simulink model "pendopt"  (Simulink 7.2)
settings: Solver=ode3  StartTime=0.0  StopTime=10  FixedStep=0.1  RelTol=1e-3
PreLoadFcn:
  | pid=readfis('pid.fis');
undefined symbols (not defined in the file or in its folder): d_val, deg, i_val, kg, m, N, p_val, s
libraries: mblibv1 x8, simulink_extras x1

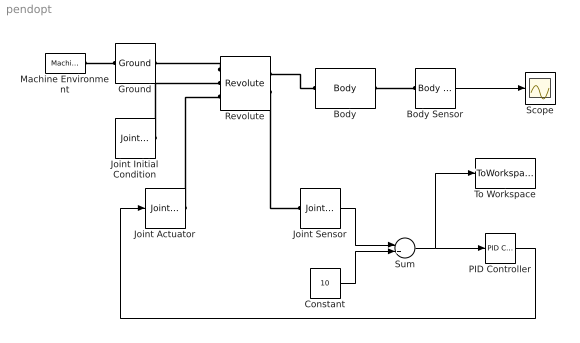
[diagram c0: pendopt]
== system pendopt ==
  Body : mblibv1/Bodies/Body  DialogController=MECH.DynMechDlgSource  PhysicalDomain=mechanical  SubClassName=Unknown  LeftPortType=workingframe  RightPortType=workingframe  LConnTagsString=CS1  RConnTagsString=CS2  UpdateFromCAD=off  DialogClass=MechanicalBodyBlock  Mass=1  MassUnits=kg  InertiaUnits=kg*m^2  Inertia=eye(3)  Shape=Cylinder  ShapeDims=[1 1]  ShapeUnits=m  ShapeUse=false  Density=1  DensityUnits=kg/m^3  DensityUse=false  GraphicsMode=MACHINE_DEFAULT  BodyColorSelMode=MACHINE_DEFAULT  BodyColor=[1 0 0]  AttachedToCS=CG  CG=Left$CG$[0 -1 0]$WORLD$WORLD$m$[0 0 0]$Euler X-Y-Z$deg$WORLD$false$none  WorkingFrames=Left$CS1$[0 0 0]$World$World$m$[0 0 0]$Euler X-Y-Z$deg$WORLD$true$none#Right$CS2$[0 -2 0]$World$World$m$[0 0 0]$Euler X-Y-Z$deg$WORLD$true$none  CGPos=[0 -1 0]  CGRot=[0 0 0]  CS0Pos=[]  CS0Rot=[]  CS1Pos=[0 0 0]  CS1Rot=[0 0 0]  CS2Pos=[0 -2 0]  CS2Rot=[0 0 0]  CS3Pos=[]  CS3Rot=[]  CS4Pos=[]  CS4Rot=[]  CS5Pos=[]  CS5Rot=[]  CS6Pos=[]  CS6Rot=[]  CS7Pos=[]  CS7Rot=[]  CS8Pos=[]  CS8Rot=[]  CS9Pos=[]  CS9Rot=[]  CS10Pos=[]  CS10Rot=[]  CS11Pos=[]  CS11Rot=[]  CS12Pos=[]  CS12Rot=[]  CS13Pos=[]  CS13Rot=[]  CS14Pos=[]  CS14Rot=[]  CS15Pos=[]  CS15Rot=[]  CS16Pos=[]  CS16Rot=[]  CS17Pos=[]  CS17Rot=[]  CS18Pos=[]  CS18Rot=[]  CS19Pos=[]  CS19Rot=[]  CS20Pos=[]  CS20Rot=[]
  Body Sensor : mblibv1/Sensors &  Actuators/Body Sensor  DialogController=MECH.DynMechDlgSource  SystemSampleTime=-1  UpdateFromCAD=off  PhysicalDomain=Mechanical  PortType=blob  Muxed=on  Pose=off  Angle=on  AngleUnits=deg  ArcVelocity=off  ArcVelocityUnits=deg/s  ArcAcceleration=off  ArcAccelerationUnits=deg/s^2  CoordPosition=on  CoordPositionUnits=m  Velocity=off  VelocityUnits=m/s  Acceleration=off  AccelerationUnits=m/s^2  Quaternion=on  QuaternionDT=off  QuaternionDDT=off  QuaternionUnits=off  OutputVector=[1]  ActiveIO=on  Width=3  DialogClass=MechanicalSensorBlock  ReferenceFrame=Absolute (World)
  Constant : Constant  Value=10  OutDataType=sfix(16)  OutScaling=2^0
  Ground : mblibv1/Bodies/Ground  DialogController=MECH.DynMechDlgSource  SystemSampleTime=-1  UpdateFromCAD=off  LeftPortType=env  RightPortType=workingframe  PhysicalDomain=Mechanical  DialogClass=GroundBlock  CoordPosition=[0 0 0]  CoordPositionUnits=m  StateVectorMgrId=-1  MachineId=[0 0]  ShowEnvPort=on
  Joint Actuator : mblibv1/Sensors &  Actuators/Joint Actuator  DialogController=MECH.DynMechDlgSource  SystemSampleTime=-1  UpdateFromCAD=off  PhysicalDomain=Mechanical  PortType=blob  ActuationStyle=Force  AngleUnits=deg  ArcVelocityUnits=deg/s  ArcAccelerationUnits=deg/s^2  CoordPositionUnits=m  VelocityUnits=m/s  AccelerationUnits=m/s^2  ForceUnits=N  TorqueUnits=N-m  ActiveIO=off  Width=1  DialogClass=MechanicalActuatorBlock  Primitive=R1  ReferenceFrame=Absolute (World)
  Joint Initial Condition : mblibv1/Sensors &  Actuators/Joint Initial Condition  DialogController=MECH.DynMechDlgSource  SystemSampleTime=-1  UpdateFromCAD=off  PhysicalDomain=mechanical  DialogClass=InitialConditionBlock  InitialConditions=P1$false$0$m$deg$0$m/s$deg/s#P2$false$0$m$deg$0$m/s$deg/s#P3$false$0$m$deg$0$m/s$deg/s#R1$true$0$m$deg$0$m/s$deg/s#R2$false$0$m$deg$0$m/s$deg/s#R3$false$0$m$deg$0$m/s$deg/s#S$false$0$m$deg$0$m/s$deg/s  P1PIC=0  P1VIC=0  P2PIC=0  P2VIC=0  P3PIC=0  P3VIC=0  R1PIC=0  R1VIC=0  R2PIC=0  R2VIC=0  R3PIC=0  R3VIC=0  SPIC=0  SVIC=0
  Joint Sensor : mblibv1/Sensors &  Actuators/Joint Sensor  DialogController=MECH.DynMechDlgSource  SystemSampleTime=-1  UpdateFromCAD=off  PhysicalDomain=Mechanical  PortType=blob  Muxed=on  Pose=off  Angle=on  AngleUnits=deg  ArcVelocity=off  ArcVelocityUnits=deg/s  ArcAcceleration=off  ArcAccelerationUnits=deg/s^2  CoordPosition=on  CoordPositionUnits=m  Velocity=off  VelocityUnits=m/s  Acceleration=off  AccelerationUnits=m/s^2  Quaternion=on  QuaternionDT=off  QuaternionDDT=off  QuaternionUnits=off  OutputVector=[1]  ActiveIO=off  Width=1  DialogClass=MechanicalSensorBlock  Primitive=R1  Force=off  ForceUnits=N  Torque=off  TorqueUnits=N-m  ReferenceFrame=Absolute (World)  ReactionSensedSide=Base  ReactionReferenceFrame=Absolute (World)  ReactionForce=off  ReactionForceUnits=N  ReactionMoment=off  ReactionMomentUnits=N-m
  Machine Environment : mblibv1/Bodies/Machine Environment  Tag=Factory ground  DialogController=MECH.DialogSource  SystemSampleTime=-1  PortType=env  PhysicalDomain=Mechanical  DialogTemplateClass=MECH.MachineEnvironment  SyncWhenCopied=off  Gravity=[0 -9.81 0]  GravityUnits=m/s^2  GravityAsSignal=off  Dimensionality=Auto-detect  AnalysisType=Forward dynamics  LinearAssemblyTolerance=1e-3  LinearAssemblyToleranceUnits=m  AngularAssemblyTolerance=1e-3  AngularAssemblyToleranceUnits=rad  ConstraintSolverType=Stabilizing  ConstraintRelTolerance=1e-4  ConstraintAbsTolerance=1e-4  UseRobustSingularityHandling=off  RedundancyAnalysisToleranceType=Automatically select tolerance  RedundancyAnalysisTolerance=1e-14  StatePerturbationType=Fixed  PerturbationSize=1e-5  VisualizeMachine=on  BodyVisualizationType=Use model default body geometries  BodyColorSelMode=Use model default  DefaultBodyColor=[1 0 0]
  PID Controller : simulink_extras/Additional Linear/PID Controller  SystemSampleTime=-1  P=p_val  I=i_val  D=d_val
  Revolute : mblibv1/Joints/Revolute  DialogController=MECH.DynMechDlgSource  PhysicalDomain=mechanical  SubClassName=Unknown  LeftPortType=blob  RightPortType=blob  LConnTagsString=__newl0|SA1|SA2  RConnTagsString=__newr0|SA1  UpdateFromCAD=off  NumSAPorts=3  CutJoint=off  MarkAsCut=off  Primitives=prismatic  PrimitiveProps=R1$World$[0 0 1]$revolute  DialogClass=JointBlock  R1Axis=[0 0 1]
  Scope : Scope
  Sum : Sum  Inputs=-+  OutDataType=sfix(16)  OutScaling=2^0
  To Workspace : ToWorkspace  VariableName=error  SampleTime=-1  SaveFormat=Structure
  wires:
  Body Sensor/1 -> Scope/1
  Joint Sensor/1 -> Sum/1
  Sum/1 -> PID Controller/1, To Workspace/1
  Constant/1 -> Sum/2
  PID Controller/1 -> Joint Actuator/1
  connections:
  Machine Environment/RConn1 -- Ground/LConn1
  Revolute/LConn1 -- Ground/RConn1
  Body/LConn1 -- Revolute/RConn1
  Body Sensor/LConn1 -- Body/RConn1
  Joint Initial Condition/RConn1 -- Revolute/LConn2
  Joint Actuator/RConn1 -- Revolute/LConn3
  Revolute/RConn2 -- Joint Sensor/LConn1
